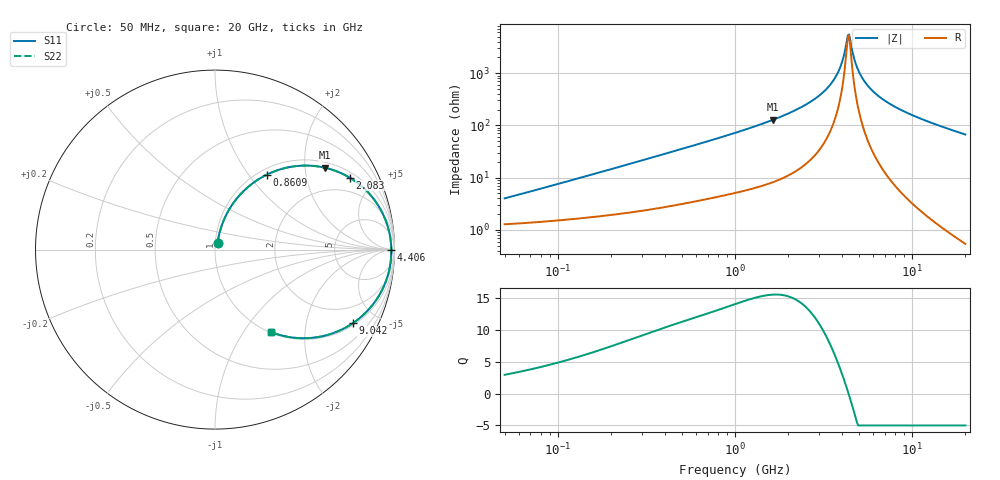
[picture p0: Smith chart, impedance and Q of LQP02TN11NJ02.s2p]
!Murata Part Number: LQP02TN11NJ02
!These Parameters are Measured in Series Mode Connection
!  o--[Z]--o
!Port1  Port2
!  o-------o
!Freq. Start=50[MHz] Stop=20[GHz], 401[Steps]
# Hz S RI R 50
!Freq.(Hz) S11(Real) S11(Imag) S21(Real) S21(Imag) S12(Real) S12(Imag) S22(Real) S22(Imag)
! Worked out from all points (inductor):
!   401 points, 50 MHz to 20 GHz, reference 50 ohm
!   read as one part in series: L = 12 nH near 51.52 MHz
!   highest Q = 15.6 at 1.639 GHz (marker M1), where L = 12.4 nH
!   self-resonance near 4.34 GHz
!   S11 on the Smith chart (normalised r, x): 50 MHz: 1.03, +0.08; 860.9 MHz: 1.09, +1.22; 2.083 GHz: 1.24, +3.59; 4.406 GHz: open; 9.042 GHz: 1.09, -3.68; 20 GHz: 1.01, -1.34
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5e7  0.0141 0.0371  0.9859 -0.0371  0.9859 -0.0371  0.0141 0.0371
1.364002e8  0.0259 0.0957  0.9741 -0.0957  0.9741 -0.0957  0.0259 0.0957
3.721004e8  0.0859 0.2351  0.9141 -0.2351  0.9141 -0.2351  0.0859 0.2351
5.831961e8  0.1652 0.3317  0.8348 -0.3317  0.8348 -0.3317  0.1652 0.3317
8.608917e8  0.2871 0.4168  0.7129 -0.4168  0.7129 -0.4168  0.2871 0.4168
1e9  0.3503 0.4429  0.6497 -0.4429  0.6497 -0.4429  0.3503 0.4429
1.639343e9  0.6139 0.4558  0.3861 -0.4558  0.3861 -0.4558  0.6139 0.4558
2.083303e9  0.7501 0.4012  0.2499 -0.4012  0.2499 -0.4012  0.7501 0.4012
2.728004e9  0.8797 0.2879  0.1203 -0.2879  0.1203 -0.2879  0.8797 0.2879
3.265178e9  0.9406 0.1877  0.0594 -0.1877  0.0594 -0.1877  0.9406 0.1877
3.680849e9  0.9669 0.1134  0.0331 -0.1134  0.0331 -0.1134  0.9669 0.1134
3.967106e9  0.977 0.0651  0.023 -0.0651  0.023 -0.0651  0.977 0.0651
4.275624e9  0.982 0.0158  0.018 -0.0158  0.018 -0.0158  0.982 0.0158
4.405649e9  0.9826 -0.00402  0.0174 0.00402  0.0174 0.00402  0.9826 -0.00402
4.472136e9  0.9826 -0.0139  0.0174 0.0139  0.0174 0.0139  0.9826 -0.0139
4.81993e9  0.9794 -0.0635  0.0206 0.0635  0.0206 0.0635  0.9794 -0.0635
5.273168e9  0.9688 -0.1224  0.0312 0.1224  0.0312 0.1224  0.9688 -0.1224
6.125241e9  0.9352 -0.2165  0.0648 0.2165  0.0648 0.2165  0.9352 -0.2165
7.442007e9  0.8638 -0.3253  0.1362 0.3253  0.1362 0.3253  0.8638 -0.3253
9.041845e9  0.7666 -0.411  0.2334 0.411  0.2334 0.411  0.7666 -0.411
1.314879e10  0.5421 -0.4915  0.4579 0.4915  0.4579 0.4915  0.5421 -0.4915
2e10  0.3104 -0.4587  0.6896 0.4587  0.6896 0.4587  0.3104 -0.4587
